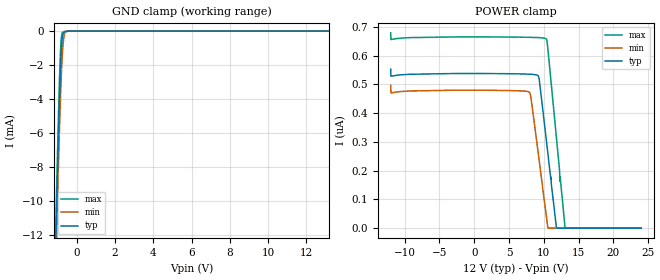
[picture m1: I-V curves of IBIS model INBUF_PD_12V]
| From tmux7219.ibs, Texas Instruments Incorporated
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| Model2
[Model]   INBUF_PD_12V
Model_type   Input
Vinl = 0.8
Vinh = 1.3
|   typ   min   max
C_comp   1.85pF   1.7pF   2.1pF
[Voltage Range]   12   10.8   13.2
[Temperature Range]   27   130   -40
[Power Clamp Reference]   12   10.8   13.2
[GND Clamp Reference]   0   0   0
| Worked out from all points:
|   GND clamp passes 1 mA (typ) near -0.80 V on its own axis
[GND Clamp]
|   Voltage   I(typ)   I(min)   I(max)
-12V      -596.9mA   -596.3mA   -597.6mA
-1.128V   -14.01mA   -15.55mA   -12.97mA
-1.092V   -12.28mA   -13.86mA   -11.2mA
-1.056V   -10.57mA   -12.2mA    -9.464mA
-1.02V    -8.907mA   -10.58mA   -7.765mA
-912mV    -4.294mA   -6.045mA   -3.1mA
-840mV    -1.878mA   -3.502mA   -895.6uA
-804mV    -1.033mA   -2.465mA   -336.6uA
-732mV    -183.9uA   -979.8uA   -62.88uA
-696mV    -130.1uA   -527.2uA   -52.34uA
-624mV    -22.62uA   -106.2uA   -31.25uA
24V       0A         0A         0A
[POWER Clamp]
|   Voltage   I(typ)   I(min)   I(max)
-12V      552.8nA    496.6nA    678.7nA
-11.96V   528.1nA    470.1nA    655.5nA
7.944V    535.1nA    471.7nA    663.2nA
9.276V    525.1nA    246.4nA    662.3nA
10.36V    307.4nA    43.78nA    657.5nA
10.57V    262.3nA    2.086nA    625.9nA
11.8V     4.862nA    0A         319.3nA
12.26V    0A         0A         200.9nA
12.3V     0A         0A         163.2nA
12.34V    0A         0A         179.2nA
13.06V    0A         0A         471pA
24V       0A         0A         0A
